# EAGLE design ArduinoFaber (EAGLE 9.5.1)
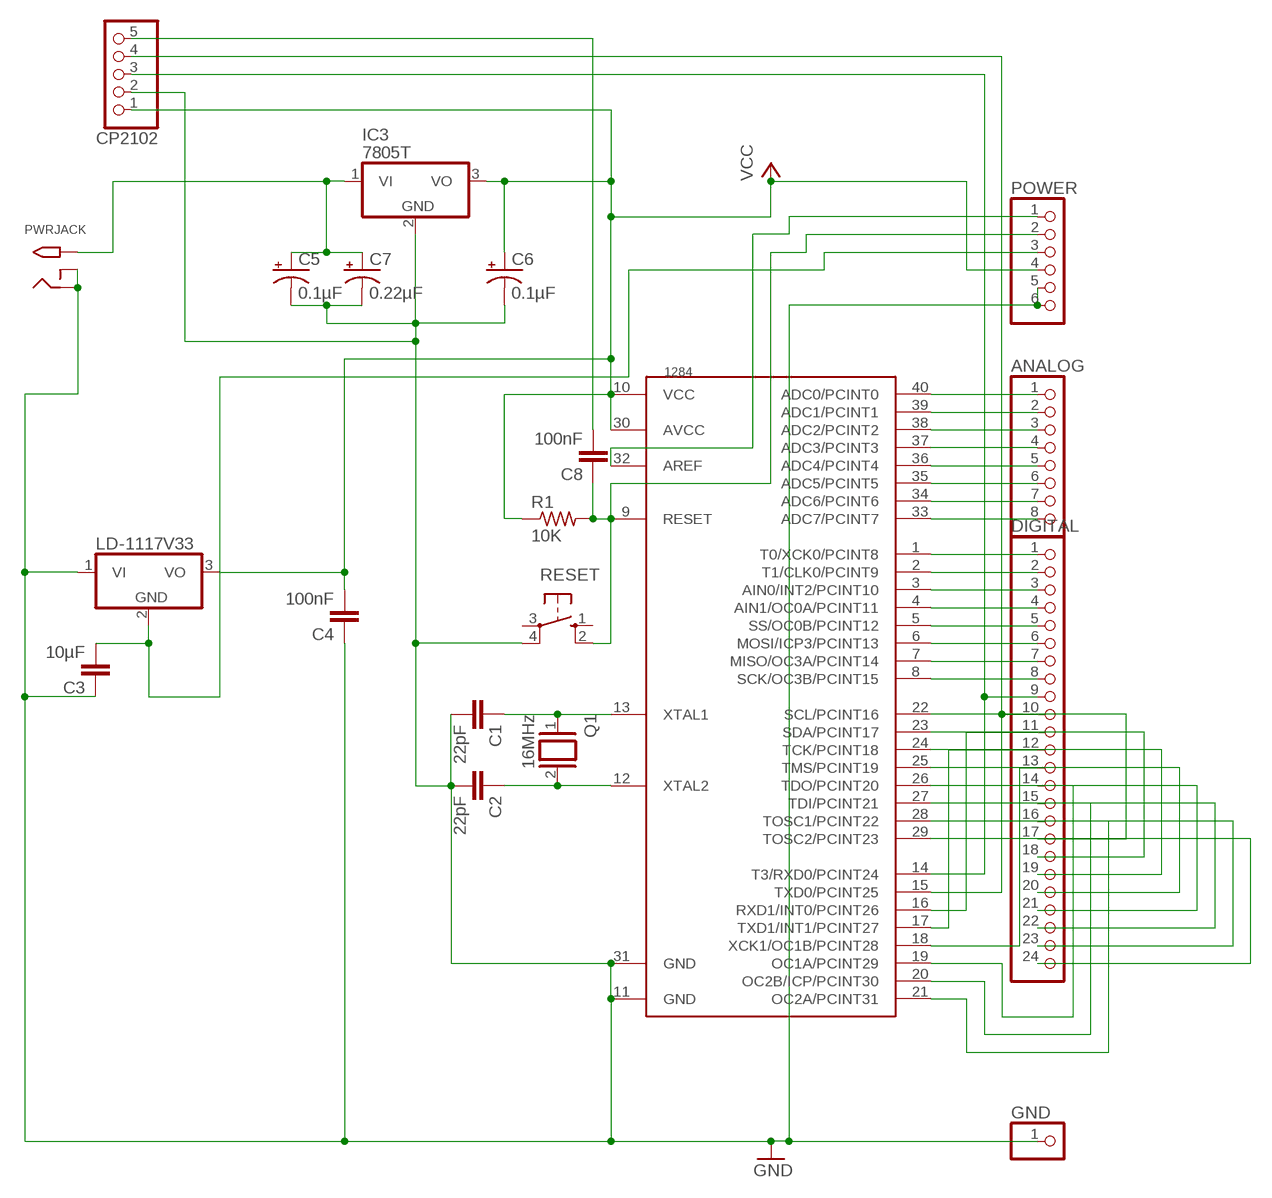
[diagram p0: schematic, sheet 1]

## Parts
1284  MEGA1284P  [DIL40]
ANALOG  PINHD-1X8  [1X08]
C1  22pF  C2.5/5  [C2.5-5]
C2  22pF  C2.5/5  [C2.5-5]
C3  10µF  C2.5/5  [C2.5-5]
C4  100nF  C2.5/5  [C2.5-5]
C5  0.1µF  CPOL-USE2-4  [E2-4]
C6  0.1µF  CPOL-USE2-4  [E2-4]
C7  0.22µF  CPOL-USE2.5-5  [E2,5-5]
C8  100nF  C2.5/5  [C2.5-5]
CP2102  PINHD-1X5  [1X05]
DIGITAL  PINHD-1X24  [1X24]
GND  PINHD-1X1  [1X01]
IC3  7805T  [TO220H]
LD-1117V33  7805T  [TO220H]
POWER  PINHD-1X6  [1X06]
PWRJACK  2.1MMJACKTHM  [PJ-102A]
Q1  16MHz  XTAL/S  [QS]
R1  10K  R-US_0207/10  [0207/10]
RESET  10-XX  [B3F-10XX]

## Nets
GND: 1284.11(GND) 1284.31(GND) C1.2 C2.2 C3.1 C4.1 C5.- C6.- C7.- CP2102.2 GND.1 IC3.2(GND) LD-1117V33.1(VI) POWER.5 POWER.6 PWRJACK.RING PWRJACK.RING_SW RESET.4(P1)
N$1: 1284.13(XTAL1) C1.1 Q1.1
N$2: 1284.12(XTAL2) C2.1 Q1.2
N$3: 1284.9(RESET) C8.1 POWER.2 R1.2 RESET.2(S1)
N$4: C3.2 LD-1117V33.2(GND) POWER.3
N$5: C8.2 CP2102.5
N$6: 1284.14(T3/RXD0/PCINT24) CP2102.3 DIGITAL.9
N$7: 1284.15(TXD0/PCINT25) CP2102.4 DIGITAL.10
N$8: 1284.40(ADC0/PCINT0) ANALOG.1
N$9: 1284.39(ADC1/PCINT1) ANALOG.2
N$10: 1284.38(ADC2/PCINT2) ANALOG.3
N$11: 1284.37(ADC3/PCINT3) ANALOG.4
N$12: 1284.36(ADC4/PCINT4) ANALOG.5
N$13: 1284.35(ADC5/PCINT5) ANALOG.6
N$14: 1284.34(ADC6/PCINT6) ANALOG.7
N$15: 1284.33(ADC7/PCINT7) ANALOG.8
N$16: 1284.32(AREF) POWER.1
N$17: 1284.1(T0/XCK0/PCINT8) DIGITAL.1
N$18: 1284.2(T1/CLK0/PCINT9) DIGITAL.2
N$19: 1284.3(AIN0/INT2/PCINT10) DIGITAL.3
N$20: 1284.4(AIN1/OC0A/PCINT11) DIGITAL.4
N$21: 1284.5(SS/OC0B/PCINT12) DIGITAL.5
N$22: 1284.6(MOSI/ICP3/PCINT13) DIGITAL.6
N$23: 1284.7(MISO/OC3A/PCINT14) DIGITAL.7
N$24: 1284.8(SCK/OC3B/PCINT15) DIGITAL.8
N$25: 1284.16(RXD1/INT0/PCINT26) DIGITAL.11
N$26: 1284.17(TXD1/INT1/PCINT27) DIGITAL.12
N$27: 1284.18(XCK1/OC1B/PCINT28) DIGITAL.13
N$28: 1284.19(OC1A/PCINT29) DIGITAL.14
N$29: 1284.20(OC2B/ICP/PCINT30) DIGITAL.15
N$30: 1284.21(OC2A/PCINT31) DIGITAL.16
N$31: 1284.22(SCL/PCINT16) DIGITAL.17
N$32: 1284.23(SDA/PCINT17) DIGITAL.18
N$33: 1284.24(TCK/PCINT18) DIGITAL.19
N$34: 1284.25(TMS/PCINT19) DIGITAL.20
N$35: 1284.26(TDO/PCINT20) DIGITAL.21
N$36: 1284.27(TDI/PCINT21) DIGITAL.22
N$37: 1284.28(TOSC1/PCINT22) DIGITAL.23
N$38: 1284.29(TOSC2/PCINT23) DIGITAL.24
N$76: C5.+ C7.+ IC3.1(VI) PWRJACK.TIP
VCC: 1284.10(VCC) 1284.30(AVCC) C4.2 C6.+ CP2102.1 IC3.3(VO) LD-1117V33.3(VO) POWER.4 R1.1
Unconnected: RESET.1(S) RESET.3(P)

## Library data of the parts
1284 = 1284p:MEGA1284P: Atmel ATmega1284P 8-bit AVR Microcontroller
ANALOG = pinhead:PINHD-1X8: PIN HEADER
C1-C4 C8 = capacitor-wima:C: CAPACITOR
C5-C7 = adafruit:CPOL-US: POLARIZED CAPACITOR, American symbol
CP2102 = pinhead:PINHD-1X5: PIN HEADER
DIGITAL = pinhead:PINHD-1X24: PIN HEADER
GND = pinhead:PINHD-1X1: PIN HEADER
IC3 LD-1117V33 = adafruit:78*: Positive VOLTAGE REGULATOR Added bigger pads to the TO-92 package
POWER = pinhead:PINHD-1X6: PIN HEADER
PWRJACK = adafruit:2.1MMJACK: 2.1mm x 5.5mm THM DC jack with internal switch. Digikey part #PJ-102A, 4UCON part #05537 2.1mm x 5.5mm SMT DC jack with internal switch. Digikey part #PJ-002A-SMT, 4UCON part #03267 By microbuilder.eu & adafruit.com
Q1 = special:XTAL/S: CRYSTAL
R1 = adafruit:R-US_: RESISTOR, American symbol
RESET = switch-omron:10-XX: OMRON SWITCH; MPN: B3F-1000; OC_FARNELL: 176432; OC_NEWARK: 36M3542

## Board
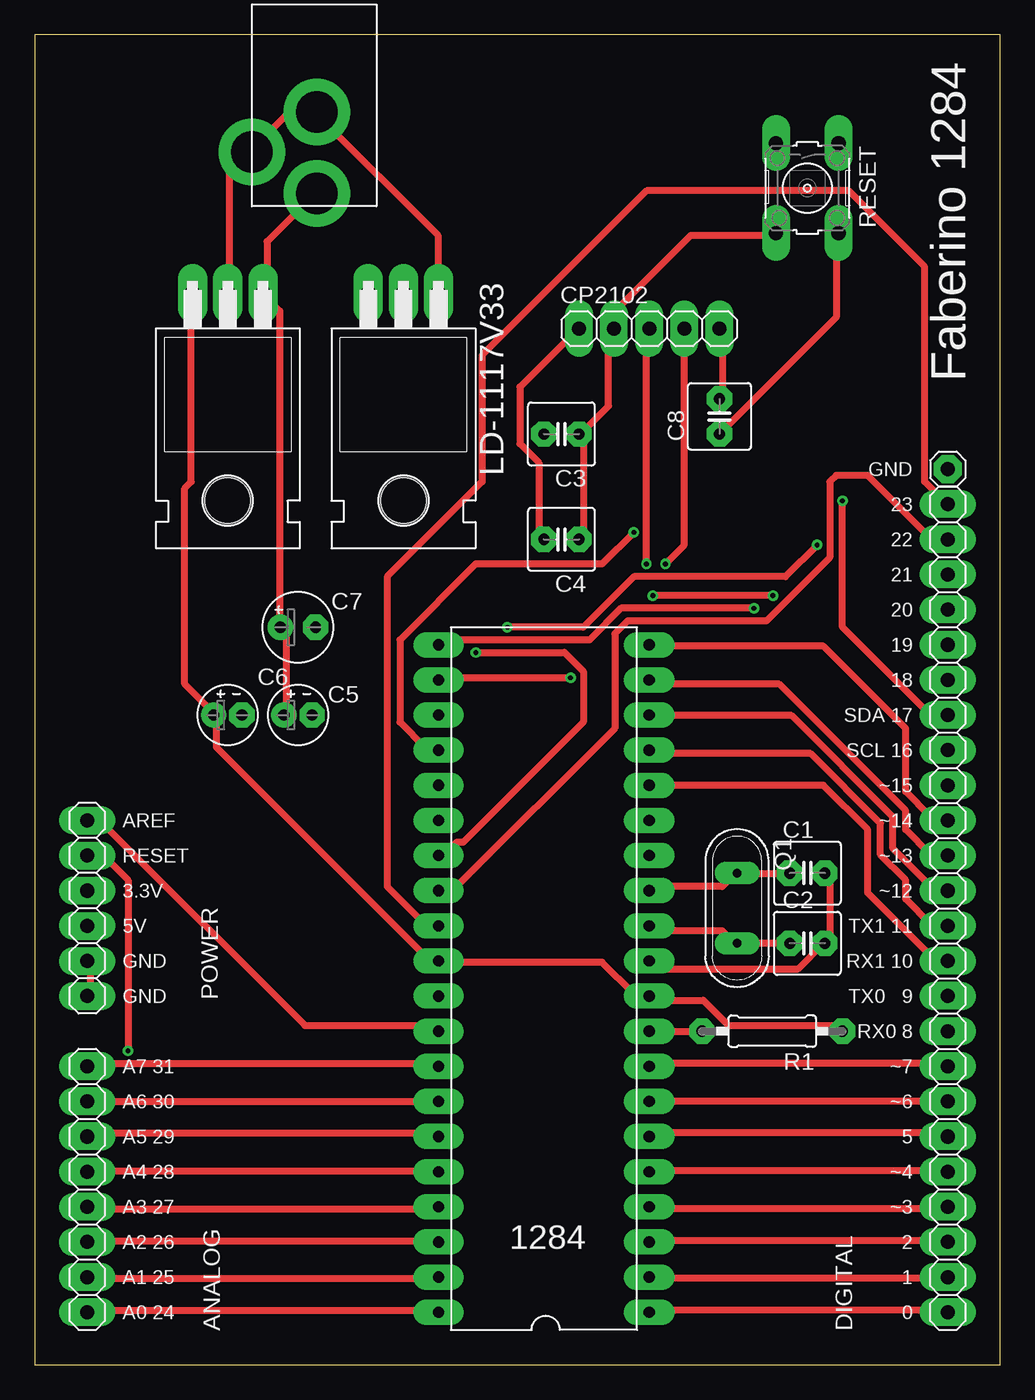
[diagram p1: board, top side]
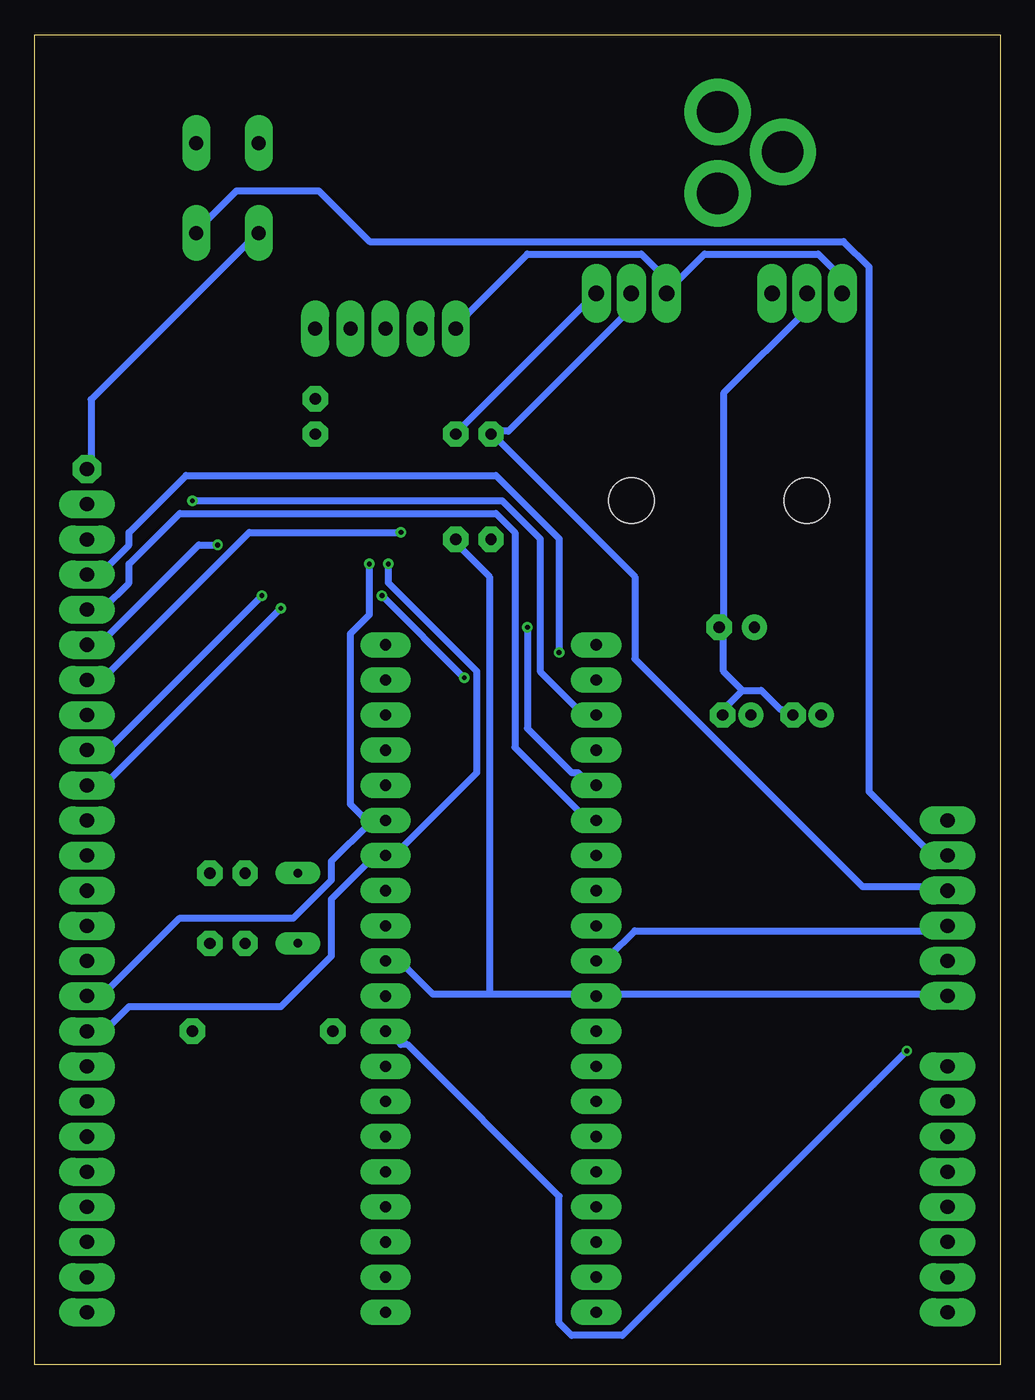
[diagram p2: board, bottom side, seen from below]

Size 69.83 x 96.19 mm. Coordinates in mm from the lower left corner, seen from the top.
Outline: 0,0 69.83,0 69.83,96.19 0,96.19 0,0
Copper layers (1*16): Top 0.035mm / dielectric 1.5mm / Bottom 0.035mm
Design rules "default *": minimum track width 20mil, minimum drill 0.35mm, track to track 16mil, track to pad 16mil, pad to pad 6mil, via to via 6mil, smd to smd 6mil, copper to edge 40mil, drill to drill 6mil, minimum pad ring 20mil, minimum via ring 8mil, stop-mask expansion 4mil, vias tented up to drill 0mil, thermal gap 10mil

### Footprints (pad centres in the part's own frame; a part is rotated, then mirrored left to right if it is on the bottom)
DIL40 = drill 0.813 long: 1 -24.13,-7.62; 2 -21.59,-7.62; 3 -19.05,-7.62; 4 -16.51,-7.62; 5 -13.97,-7.62; 6 -11.43,-7.62; 7 -8.89,-7.62; 8 -6.35,-7.62; 9 -3.81,-7.62; 10 -1.27,-7.62; 11 1.27,-7.62; 12 3.81,-7.62; 13 6.35,-7.62; 14 8.89,-7.62; 15 11.43,-7.62; 16 13.97,-7.62; 17 16.51,-7.62; 18 19.05,-7.62; 19 21.59,-7.62; 20 24.13,-7.62; 21 24.13,7.62; 22 21.59,7.62; 23 19.05,7.62; 24 16.51,7.62; 25 13.97,7.62; 26 11.43,7.62; 27 8.89,7.62; 28 6.35,7.62; 29 3.81,7.62; 30 1.27,7.62; 31 -1.27,7.62; 32 -3.81,7.62; 33 -6.35,7.62; 34 -8.89,7.62; 35 -11.43,7.62; 36 -13.97,7.62; 37 -16.51,7.62; 38 -19.05,7.62; 39 -21.59,7.62; 40 -24.13,7.62
1X08 = drill 1.016 long: 1 -8.89,0; 2 -6.35,0; 3 -3.81,0; 4 -1.27,0; 5 1.27,0; 6 3.81,0; 7 6.35,0; 8 8.89,0
C2.5-5 = drill 0.813 pad 1.6 octagon: 1 -1.27,0; 2 1.27,0
E2-4 = drill 0.813 pad 1.422: + -1.016,0 | drill 0.813 pad 1.422 octagon: - 1.016,0
E2,5-5 = drill 0.813 pad 1.6: + -1.27,0 | drill 0.813 pad 1.6 octagon: - 1.27,0
1X05 = drill 1.016 long: 1 -5.08,0; 2 -2.54,0; 3 0,0; 4 2.54,0; 5 5.08,0
1X24 = drill 1.016 long: 1 -29.21,0; 2 -26.67,0; 3 -24.13,0; 4 -21.59,0; 5 -19.05,0; 6 -16.51,0; 7 -13.97,0; 8 -11.43,0; 9 -8.89,0; 10 -6.35,0; 11 -3.81,0; 12 -1.27,0; 13 1.27,0; 14 3.81,0; 15 6.35,0; 16 8.89,0; 17 11.43,0; 18 13.97,0; 19 16.51,0; 20 19.05,0; 21 21.59,0; 22 24.13,0; 23 26.67,0; 24 29.21,0
1X01 = drill 1.016 octagon: 1 0,0
TO220H = drill 1.118 long: 1 -2.54,-10.16; 2 0,-10.16; 3 2.54,-10.16 | hole 3.302: 0,4.826
1X06 = drill 1.016 long: 1 -6.35,0; 2 -3.81,0; 3 -1.27,0; 4 1.27,0; 5 3.81,0; 6 6.35,0
PJ-102A = drill 3 pad 4.8: RING 0.1,-3.39; RING_SW -4.6,-6.29; TIP 0.1,-9.29
QS = drill 0.61 long: 1 -2.54,0; 2 2.54,0
0207/10 = drill 0.813 pad 1.676 octagon: 1 -5.08,0; 2 5.08,0
B3F-10XX = drill 1.016 long: 1 -3.251,2.261; 2 3.251,2.261; 3 -3.251,-2.261; 4 3.251,-2.261

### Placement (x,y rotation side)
1284  36.83,27.94 90 top
ANALOG  3.81,12.7 90 top
C1  55.88,35.56 0 top
C2  55.88,30.48 0 top
C3  38.1,67.31 180 top
C4  38.1,59.69 180 top
C5  19.05,46.99 0 top
C6  13.97,46.99 0 top
C7  19.05,53.34 0 top
C8  49.53,68.58 90 top
CP2102  44.45,74.93 0 top
DIGITAL  66.04,33.02 90 top
GND  66.04,64.77 0 top
IC3  13.97,67.31 180 top
LD-1117V33  26.67,67.31 180 top
POWER  3.81,33.02 270 top
PWRJACK  20.32,93.98 0 top
Q1  50.8,33.02 270 top
R1  53.34,24.13 180 top
RESET  55.88,85.09 270 top

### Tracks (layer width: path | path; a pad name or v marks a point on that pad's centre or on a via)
GND
  Top 0.508: C1.2 57.51,35.51 57.51,30.48 C2.2 57.05,30.48 55.22,28.65 45.16,28.65 44.7,29.11 1284.11 | POWER.6 4.01,26.82 4.01,29.11 POWER.5 | C4.1 39.68,59.74 39.68,67.06 C3.1 39.68,67.51 41.5,69.34 41.5,74.83 CP2102.2 41.96,75.29 41.96,76.2 47.45,81.69 53.39,81.69 RESET.4 | IC3.2 14.07,77.57 14.07,86.26 15.44,87.63 PWRJACK.RING_SW 15.9,88.09 18.19,90.37 20.02,90.37 PWRJACK.RING 20.47,90.37 29.16,81.69 29.16,77.57 LD-1117V33.1
  Bottom 0.508: 36.93,26.82 41.05,26.82 43.33,29.11 44.25,29.11 1284.11 | 36.93,26.82 29.62,26.82 1284.31 29.16,26.82 4.01,26.82 POWER.6 | GND.1 65.73,64.77 65.73,69.8 53.85,81.69 RESET.4 | LD-1117V33.1 29.62,77.11 39.22,67.51 C3.1 | 18.64,48.77 17.27,48.77 15.9,47.4 14.99,47.4 C6.- | 18.64,48.77 20.02,47.4 C5.- | 20.02,53.34 20.02,50.14 18.64,48.77 | 20.02,53.34 20.02,70.26 14.07,76.2 14.07,77.11 IC3.2 | 20.02,53.34 C7.- | 36.93,26.82 36.93,57 39.22,59.28 C4.1
N$1
  Top 0.508: C1.1 54.3,35.51 51.11,35.51 Q1.1 50.65,35.51 49.73,34.59 44.7,34.59 1284.13
N$2
  Top 0.508: C2.1 Q1.2 50.65,30.48 49.73,31.39 44.7,31.39 1284.12
N$3  (via drill 0.35)
  Top 0.508: 1284.9 44.7,24.08 47.9,24.08 R1.2 | C8.1 57.96,75.74 57.96,81.69 RESET.2 | v6.76,22.71 6.76,35.05 5.38,36.42 4.01,36.42 POWER.2
  Bottom 0.508: POWER.2 4.01,36.88 4.93,36.88 9.5,41.45 9.5,79.4 11.33,81.23 45.62,81.23 49.28,84.89 55.22,84.89 57.96,82.14 RESET.2 | v6.76,22.71 27.33,2.13 30.99,2.13 31.9,3.05 31.9,12.19 42.88,23.17 43.33,23.17 44.25,24.08 1284.9
N$4
  Bottom 0.508: LD-1117V33.2 26.87,77.11 26.87,76.2 35.56,67.51 36.47,67.51 C3.2 36.47,67.06 26.42,57 26.42,51.05 9.96,34.59 4.01,34.59 POWER.3
N$5
  Top 0.508: C8.2 49.73,70.26 49.73,74.83 CP2102.5
N$6  (via drill 0.35)
  Top 0.508: v44.25,57.91 44.25,74.83 CP2102.3
  Bottom 0.508: DIGITAL.9 65.73,24.54 64.36,24.54 62.99,25.91 52.02,25.91 48.36,29.57 48.36,33.68 45.62,36.42 44.7,36.42 1284.14 44.25,36.42 37.85,42.82 37.85,50.14 44.25,56.54 v44.25,57.91
N$7  (via drill 0.35)
  Top 0.508: CP2102.4 46.99,59.28 v45.62,57.91
  Bottom 0.508: 45.62,39.17 44.7,39.17 1284.15 45.62,39.17 | 45.62,39.17 48.36,36.42 48.36,35.05 51.11,32.31 59.33,32.31 64.82,26.82 65.73,26.82 DIGITAL.10 | v45.62,57.91 45.62,54.25 46.99,52.88 46.99,40.54 45.62,39.17
N$8
  Top 0.508: 1284.40 29.16,3.96 4.01,3.96 ANALOG.1
N$9
  Top 0.508: 1284.39 29.16,6.25 4.01,6.25 ANALOG.2
N$10
  Top 0.508: 1284.38 29.16,8.99 4.01,8.99 ANALOG.3
N$11
  Top 0.508: 1284.37 29.16,11.28 4.01,11.28 ANALOG.4
N$12
  Top 0.508: 1284.36 29.16,14.02 4.01,14.02 ANALOG.5
N$13
  Top 0.508: 1284.35 29.16,16.76 4.01,16.76 ANALOG.6
N$14
  Top 0.508: ANALOG.7 1284.34
N$15
  Top 0.508: 1284.33 29.16,21.79 4.01,21.79 ANALOG.8
N$16
  Top 0.508: 1284.32 29.16,24.54 19.56,24.54 4.93,39.17 4.01,39.17 POWER.1
N$17
  Top 0.508: 1284.1 44.7,3.96 65.73,3.96 DIGITAL.1
N$18
  Top 0.508: 1284.2 44.7,6.25 65.73,6.25 DIGITAL.2
N$19
  Top 0.508: 1284.3 44.7,8.99 65.73,8.99 DIGITAL.3
N$20
  Top 0.508: 1284.4 44.7,11.28 65.73,11.28 DIGITAL.4
N$21
  Top 0.508: 1284.5 44.7,14.02 65.73,14.02 DIGITAL.5
N$22
  Top 0.508: 1284.6 44.7,16.76 65.73,16.76 DIGITAL.6
N$23
  Top 0.508: DIGITAL.7 1284.7
N$24
  Top 0.508: 1284.8 44.7,21.79 65.73,21.79 DIGITAL.8
N$25
  Top 0.508: 1284.16 57.05,41.91 60.25,38.71 60.25,34.14 64.82,29.57 65.73,29.57 DIGITAL.11
N$26
  Top 0.508: 1284.17 44.7,44.2 56.13,44.2 61.16,39.17 61.16,36.88 62.99,35.05 62.99,33.68 64.82,31.85 65.73,31.85 DIGITAL.12
N$27
  Top 0.508: 1284.18 44.7,46.94 54.76,46.94 62.08,39.62 62.08,37.34 64.82,34.59 65.73,34.59 DIGITAL.13
N$28
  Top 0.508: 1284.19 44.7,49.22 53.85,49.22 62.99,40.08 62.99,38.71 64.82,36.88 65.73,36.88 DIGITAL.14
N$29
  Top 0.508: 1284.20 44.7,51.97 57.05,51.97 62.99,46.02 62.99,41.45 64.82,39.62 65.73,39.62 DIGITAL.15
N$30  (via drill 0.35)
  Top 0.508: v52.02,54.71 42.42,54.71 40.13,52.43 29.62,52.43 1284.21
  Bottom 0.508: v52.02,54.71 64.82,41.91 DIGITAL.16
N$31  (via drill 0.35)
  Top 0.508: v38.76,49.68 29.62,49.68 1284.22 | v53.39,55.63 v44.7,55.63
  Bottom 0.508: v44.7,55.63 v38.76,49.68 | v53.39,55.63 64.36,44.65 65.73,44.65 DIGITAL.17
N$32  (via drill 0.35)
  Top 0.508: v58.42,62.48 58.42,53.34 64.36,47.4 65.73,47.4 DIGITAL.18
  Bottom 0.508: v58.42,62.48 36.02,62.48 33.27,59.74 33.27,50.14 30.53,47.4 29.62,47.4 1284.23
N$33  (via drill 0.35)
  Top 0.508: v43.33,60.2 41.05,57.91 31.9,57.91 26.42,52.43 26.42,46.48 28.25,44.65 29.16,44.65 1284.24
  Bottom 0.508: v43.33,60.2 54.3,60.2 64.82,49.68 65.73,49.68 DIGITAL.19
N$34  (via drill 0.35)
  Top 0.508: v34.19,53.34 39.68,53.34 43.33,57 54.3,57 v56.59,59.28
  Bottom 0.508: v34.19,53.34 34.19,46.02 30.99,42.82 30.53,42.82 29.62,41.91 1284.25 | v56.59,59.28 57.96,59.28 64.82,52.43 65.73,52.43 DIGITAL.20
N$35
  Bottom 0.508: 1284.26 29.62,39.62 30.07,39.62 35.1,44.65 35.1,60.2 36.47,61.57 59.33,61.57 62.99,57.91 62.99,56.54 64.82,54.71 65.73,54.71 DIGITAL.21
N$36  (via drill 0.35)
  Top 0.508: v31.9,51.51 38.3,51.51 39.68,50.14 39.68,46.48 30.99,37.79 30.53,37.79 29.62,36.88 1284.27
  Bottom 0.508: v31.9,51.51 31.9,59.74 36.47,64.31 58.88,64.31 62.99,60.2 62.99,59.28 64.82,57.45 65.73,57.45 DIGITAL.22
N$37
  Top 0.508: 1284.28 29.62,34.59 30.53,34.59 41.96,46.02 41.96,52.88 42.88,53.8 52.93,53.8 57.51,58.37 57.51,63.86 57.96,64.31 60.25,64.31 64.82,59.74 65.73,59.74 DIGITAL.23
N$38
  Top 0.508: 1284.29 29.16,31.85 28.25,31.85 25.5,34.59 25.5,57 32.36,63.86 32.36,73 44.25,84.89 58.88,84.89 64.36,79.4 64.36,63.86 65.73,62.48 DIGITAL.24
N$76
  Top 0.508: C5.+ 18.19,47.4 18.19,53.34 C7.+ 17.73,53.34 17.73,76.2 16.82,77.11 IC3.1 16.82,77.57 16.82,81.23 20.02,84.43 PWRJACK.TIP
VCC
  Top 0.508: C4.2 36.47,59.74 36.47,65.23 35.1,66.6 35.1,70.71 39.22,74.83 CP2102.1 | R1.1 58.42,24.54 50.19,24.54 48.36,26.37 44.7,26.37 1284.10 44.25,26.82 43.33,26.82 41.05,29.11 29.62,29.11 1284.30 29.16,29.57 28.25,29.57 13.16,44.65 13.16,46.94 C6.+ 12.7,47.4 10.87,49.22 10.87,63.4 11.33,63.86 11.33,77.11 IC3.3
  Bottom 0.508: 23.67,78.03 24.13,77.57 LD-1117V33.3 23.67,78.03 | 23.67,78.03 21.39,80.31 13.16,80.31 11.79,78.94 11.79,77.57 IC3.3 | 23.67,78.03 25.96,80.31 34.19,80.31 39.22,75.29 CP2102.1 | POWER.4 4.01,31.39 26.42,31.39 28.25,29.57 29.16,29.57 1284.30

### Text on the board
tNames: Faberino 1284 | GND | 23 | 22 | 21 | 20 | 19 | 18 | SDA 17 | SCL 16 | ~15 | AREF | ~14 | RESET | ~13 | 3.3V | ~12 | 5V | TX1 11 | GND | RX1 10 | GND | TX0 9 | RX0 8 | A7 31 | ~7 | A6 30 | ~6 | A5 29 | 5 | A4 28 | ~4 | A3 27 | ~3 | A2 26 | 2 | A1 25 | 1 | A0 24 | 0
